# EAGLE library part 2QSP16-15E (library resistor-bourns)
BOURNS RESISTOR NETWORK
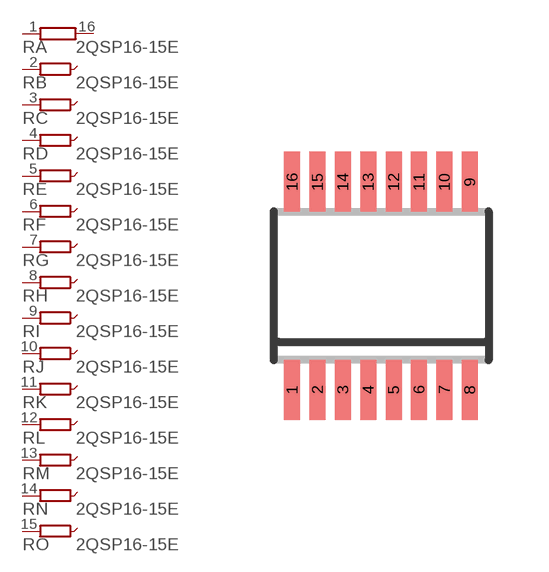
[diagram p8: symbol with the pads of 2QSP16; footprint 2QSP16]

Designator prefix R; gates A=R1NV B=R1NVXX C=R1NVXX D=R1NVXX E=R1NVXX F=R1NVXX G=R1NVXX H=R1NVXX I=R1NVXX J=R1NVXX K=R1NVXX L=R1NVXX M=R1NVXX N=R1NVXX O=R1NVXX

## 2QSP16-15E (OC_FARNELL: unknown; OC_NEWARK: unknown)  [2QSP16]
1  A:1  pas
2  B:1  pas
3  C:1  pas
4  D:1  pas
5  E:1  pas
6  F:1  pas
7  G:1  pas
8  H:1  pas
9  I:1  pas
10  J:1  pas
11  K:1  pas
12  L:1  pas
13  M:1  pas
14  N:1  pas
15  O:1  pas
16  A:2  pas

## Footprint 2QSP16 (pad centres in mm)
BOURNS RESISTOR NETWORK
smd 0.4 x 1.5: 1 -2.223,-2.6; 2 -1.588,-2.6; 3 -0.953,-2.6; 4 -0.318,-2.6; 5 0.318,-2.6; 6 0.953,-2.6; 7 1.588,-2.6; 8 2.223,-2.6; 9 2.223,2.6; 10 1.588,2.6; 11 0.953,2.6; 12 0.318,2.6; 13 -0.318,2.6; 14 -0.953,2.6; 15 -1.588,2.6; 16 -2.223,2.6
